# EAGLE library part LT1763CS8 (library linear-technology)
500mA, Low Noise, LDO Micropower Regulators Source: http://cds.linear.com/docs/Datasheet/1763ff.pdf
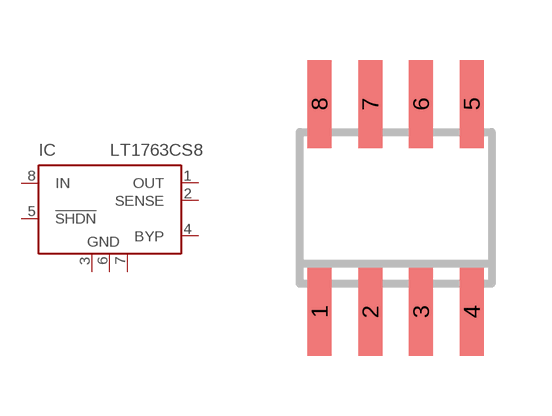
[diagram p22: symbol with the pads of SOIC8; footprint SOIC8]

Designator prefix IC

## LT1763CS8-1.5 (MPN: LT1763CS8-1.5; OC_FARNELL: 1501016; OC_NEWARK: 57M6043), LT1763CS8-1.8 (MPN: LT1763CS8-1.8; OC_FARNELL: 1273615; OC_NEWARK: 57M6047), LT1763CS8-2.5 (MPN: LT1763CS8-2.5; OC_FARNELL: 1273616; OC_NEWARK: 57M6051), LT1763CS8-3 (MPN: LT1763CS8-3; OC_FARNELL: unknown; OC_NEWARK: 02E0014), LT1763CS8-3.3 (MPN: LT1763CS8-3.3; OC_FARNELL: 1273617; OC_NEWARK: 57M6055)  [SOIC8]
1  OUT  pas
2  SENSE  in
3  GND  pwr
4  BYP  in
5  !SHDN  in
6  GND  pwr
7  GND  pwr
8  IN  in

## Footprint SOIC8 (pad centres in mm)
Small Outline IC
smd 0.6 x 2.2: 1 -1.905,-2.6; 2 -0.635,-2.6; 3 0.635,-2.6; 4 1.905,-2.6; 5 1.905,2.6; 6 0.635,2.6; 7 -0.635,2.6; 8 -1.905,2.6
